// ***************************************************************************
// UDT986

// Datum	  Name	Aktion
// ---------------------------------------------------------------------------
// 29.10.97   Mahler	Neu

TYPE "XC_BUFF_SR_UDT"	// User-Auftrag fuer Send/Receive Schnittstelle

STRUCT


	bCRecv		: BYTE	:= B#16#0;		//Sendezaehler
	bCSend		: BYTE	:= B#16#0;		//Zaehler beim Senden erhoehen

	bDestTyp		: BYTE;				//Send:50=DB 51=DX  Fetch:52=DB 53=DX  68=PUT_Time
	bSrcTyp		: BYTE;				//
	iDBNr			: INT;				//
	iDWNr			: INT;				//
      iLen			: INT;				//Anzahl Bytes max. 104

	iDW			: ARRAY[1..114]of INT;		//Nutzdaten

      iEnd			: WORD		:= W#16#FFFF;		//Endekennung dh. -1

END_STRUCT ;

END_TYPE


